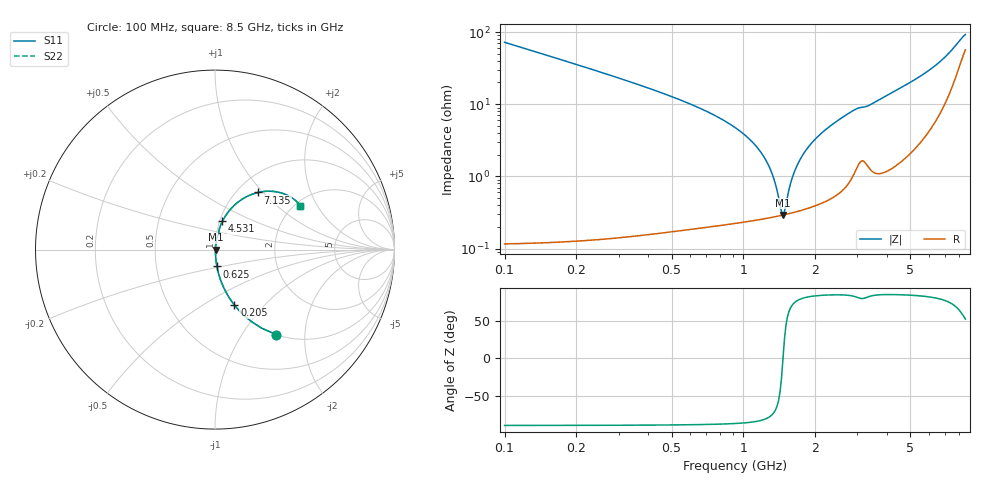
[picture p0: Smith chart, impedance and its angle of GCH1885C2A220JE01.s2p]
!Murata Part Number: GCH1885C2A220JE01
!These Parameters are Measured in Series Mode Connection
!Data Generated on Mar 13, 2026
!  o--ll--o
!Port1  Port2
!  o------o
!Operation Temp=25[degC], DC Bias Voltage=0[V]
!Freq. Start=100[MHz] Stop=9[GHz] 401[Steps]
# Hz S RI R 50
!Freq.(Hz) S11(Real) S11(Imag) S21(Real) S21(Imag) S12(Real) S12(Imag) S22(Real) S22(Imag)
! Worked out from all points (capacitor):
!   401 points, 100 MHz to 8.5 GHz, reference 50 ohm
!   read as one part in series: C = 22 pF near 142 MHz
!   lowest |Z| = 292 mohm at 1.465 GHz (marker M1)
!   series resonance near 1.465 GHz, so ESL is about 540 pH
!   S11 on the Smith chart (normalised r, x): 100 MHz: 1.00, -1.44; 205 MHz: 1.00, -0.69; 625 MHz: 1.00, -0.19; 4.531 GHz: 1.03, +0.33; 7.135 GHz: 1.24, +0.94; 8.5 GHz: 2.13, +1.46
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1e8  0.3416 -0.4735  0.6584 0.4735  0.6584 0.4735  0.3416 -0.4735
2.05e8  0.1077 -0.3082  0.8923 0.3082  0.8923 0.3082  0.1077 -0.3082
3.73e8  0.0332 -0.175  0.9668 0.175  0.9668 0.175  0.0332 -0.175
6.25e8  0.0107 -0.0935  0.9893 0.0935  0.9893 0.0935  0.0107 -0.0935
9.82e8  0.00395 -0.0406  0.9961 0.0406  0.9961 0.0406  0.00395 -0.0406
1.171e9  0.00302 -0.0224  0.997 0.0224  0.997 0.0224  0.00302 -0.0224
1.297e9  0.00283 -0.0121  0.9972 0.0121  0.9972 0.0121  0.00283 -0.0121
1.423e9  0.00286 -0.00289  0.9971 0.00289  0.9971 0.00289  0.00286 -0.00289
1.465e9  0.00291 2.23e-05  0.9971 -2.23e-05  0.9971 -2.23e-05  0.00291 2.23e-05
1.507e9  0.00298 0.00286  0.997 -0.00286  0.997 -0.00286  0.00298 0.00286
1.591e9  0.00318 0.00834  0.9968 -0.00834  0.9968 -0.00834  0.00318 0.00834
1.654e9  0.00336 0.0123  0.9966 -0.0123  0.9966 -0.0123  0.00336 0.0123
1.759e9  0.00375 0.0187  0.9963 -0.0187  0.9963 -0.0187  0.00375 0.0187
1.906e9  0.00444 0.0272  0.9956 -0.0272  0.9956 -0.0272  0.00444 0.0272
2.305e9  0.00722 0.0489  0.9928 -0.0489  0.9928 -0.0489  0.00722 0.0489
2.914e9  0.0175 0.0804  0.9825 -0.0804  0.9825 -0.0804  0.0175 0.0804
4.3e9  0.035 0.1442  0.965 -0.1442  0.965 -0.1442  0.035 0.1442
4.531e9  0.0411 0.1572  0.9589 -0.1572  0.9589 -0.1572  0.0411 0.1572
5.707e9  0.0913 0.2304  0.9087 -0.2304  0.9087 -0.2304  0.0913 0.2304
7.114e9  0.2361 0.3174  0.7639 -0.3174  0.7639 -0.3174  0.2361 0.3174
7.135e9  0.2394 0.3182  0.7606 -0.3182  0.7606 -0.3182  0.2394 0.3182
8.5e9  0.4757 0.2444  0.5243 -0.2444  0.5243 -0.2444  0.4757 0.2444
